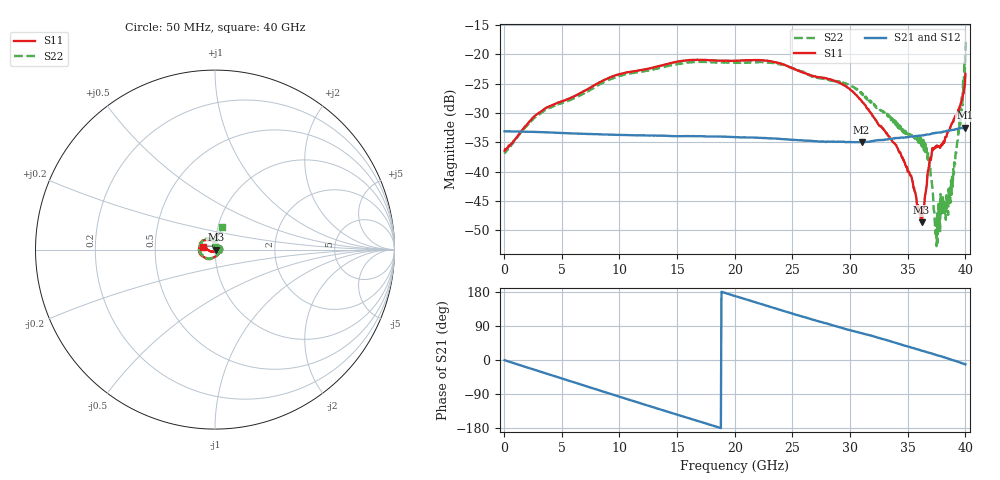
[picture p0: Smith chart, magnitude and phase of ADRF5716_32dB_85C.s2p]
! Device: ADRF5716
! Description: 30GHz 2-Bit Digital Attenuator
! Frequency: 100 MHz – 30 GHz
! Ports:
! ATTIN  = Port 1
! ATTOUT = Port 2
! State: 32 dB Attenuation selected
! Supply Voltage:
! VDD  =  +3.30 Volts
! VSS  =  -3.30 Volts
! Control Voltages:
! D5 = 0V, D6 = 3.3V
! Temperature = +85 C
! Data: Data was collected using a calibrated network analyzer.
!  The reference plane is the package pins of ADRF5716 switch.
! Note: Analog Devices supplies this data as a sample of measured data for this product.
!  Your particular data for this product may vary.
!  Analog Devices reserves the right to change this data at anytime
# HZ S DB R 50
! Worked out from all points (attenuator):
!   800 points, 50 MHz to 40 GHz, reference 50 ohm
!   highest |S21| = -32.50 dB at 39.95 GHz (marker M1); lowest = -35.0 dB at 31 GHz (marker M2)
!   lowest |S11| = -48.6 dB at 36.2 GHz (marker M3), VSWR 1.01, Z = 50.4 - j0.0471 ohm
!   |S11| at or under -10 dB: start of sweep to end of sweep
!   |S22| runs from -52.7 to -17.6 dB; largest |S21 - S12| = 0
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5e7  -36.41 5.9  -33.11 -0.5  -33.11 -0.5  -36.91 4.4
2.8e9  -30.29 -52.7  -33.23 -27.5  -33.23 -27.5  -30.48 -52.1
6.75e9  -26.46 -103.2  -33.53 -65.5  -33.53 -65.5  -26.87 -104.0
1.34e10  -22.00 -152.4  -33.83 -129.2  -33.83 -129.2  -22.36 -155.2
2.005e10  -21.10 168.4  -34.11 168.5  -34.11 168.5  -21.41 162.8
2.4e10  -21.57 142.6  -34.42 131.8  -34.42 131.8  -21.65 136.5
2.67e10  -23.65 129.6  -34.75 107.1  -34.75 107.1  -23.80 117.8
2.91e10  -24.88 113.7  -34.90 86.4  -34.90 86.4  -24.64 103.2
3.1e10  -27.95 95.6  -34.98 70.6  -34.98 70.6  -26.78 81.0
3.335e10  -33.97 89.1  -34.42 51.0  -34.42 51.0  -30.65 61.6
3.515e10  -40.17 78.7  -34.06 34.4  -34.06 34.4  -33.79 42.6
3.62e10  -48.64 -7.3  -33.83 24.9  -33.83 24.9  -35.63 23.1
3.665e10  -42.27 -77.9  -33.67 21.0  -33.67 21.0  -36.01 5.7
3.695e10  -37.64 -110.6  -33.60 18.4  -33.60 18.4  -39.25 -5.6
3.74e10  -35.99 -138.2  -33.37 14.1  -33.37 14.1  -50.61 -42.9
3.76e10  -35.69 -147.0  -33.35 12.0  -33.35 12.0  -52.08 5.6
3.785e10  -35.71 -146.5  -33.30 9.6  -33.30 9.6  -43.79 73.9
3.83e10  -34.11 -151.2  -33.11 5.6  -33.11 5.6  -48.17 22.7
3.88e10  -31.91 -157.6  -32.91 0.7  -32.91 0.7  -43.91 62.1
3.955e10  -28.80 -175.1  -32.60 -6.7  -32.60 -6.7  -32.00 114.1
3.995e10  -25.31 170.3  -32.50 -11.0  -32.50 -11.0  -23.07 85.8
4e10  -23.34 169.5  -32.59 -11.4  -32.59 -11.4  -17.65 72.3
